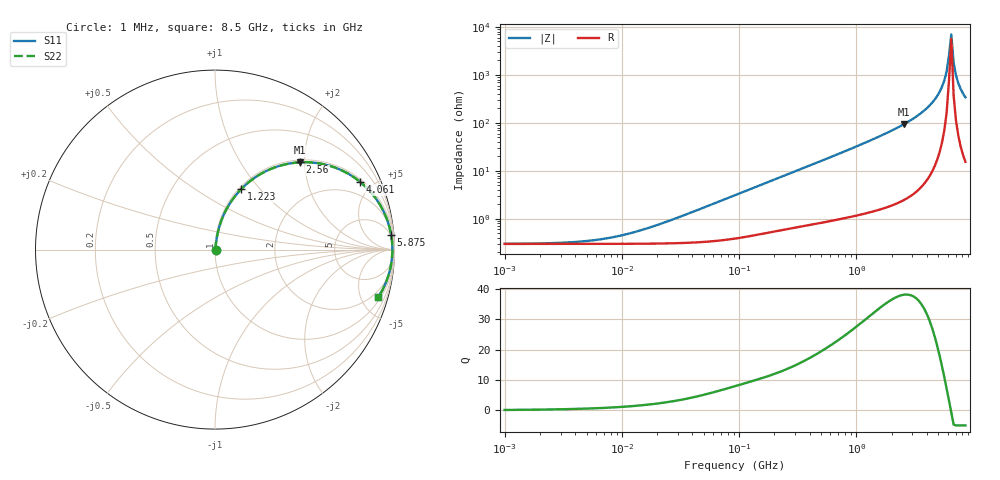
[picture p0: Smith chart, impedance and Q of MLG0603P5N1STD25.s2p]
! S-Parameter Data Generated by TDK Corporation
! Copyright(C) 2025 TDK Corporation.
! All Rights Reserved.
! TDK P/N: MLG0603P5N1STD25 (SMD / SMT Inductor (Coil))
! Property: L=5.1nH at 500MHz
! Size(LxWxT): 0.6x0.3x0.3mm
! Model Type: s2p (Touchstone File Format Version 1.0)
! Frequency: DC=Yes Start=1MHz Stop=8500MHz 198points Log-sweep
! Model Generated on Feb. 6, 2025
! Terms and conditions regarding TDK Simulation Models:
! 1)This simulation model is being provided solely for informational
!  purposes. Please refer to the specifications of the products in
!  terms of detailed characteristics of such products.
! 2)In no event shall TDK Corporation of any of its subsidiaries be
!  liable for any loss or damage arising, directly or indirectly,
!  from any information contained in this simulation model, including,
!  but not limited to loss or damages arising from any inaccuracies,
!  omissions or errors in connection with such information.
! 3)Any and all copyrights on this simulation model are owned by
!  TDK Corporation.  Duplication or redistribution of this simulation
!  model without prior written permission from TDK Corporation
!  is prohibited.
! 4)This simulation model is subject to any modification or change
!  without any prior notice.
! 5)Neither TDK Corporation nor any of its subsidiaries shall make any
!  warranty, express or implied, including but not limited to the
!  correctness, implied warranties of merchantability and fitness for
!  a particular purpose with respect to this simulation models.
! 6)The use of this simulation model shall be deemed to have consented
!  to the terms and conditions hereof.
! Port Assignments:
!  1 ---@@@--- 2
! Applicable Conditions:
!  Temperature = 25 degC
!  DC Bias Current = 0 A
!  Small Signal Operation
# Hz S MA R 50
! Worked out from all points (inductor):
!   197 points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, 1 MHz to 8.5 GHz, reference 50 ohm
!   read as one part in series: L = 5.38 nH near 27.76 MHz
!   highest Q = 38.1 at 2.56 GHz (marker M1), where L = 5.89 nH
!   self-resonance near 6.153 GHz
!   S11 on the Smith chart (normalised r, x): 1 MHz: 1.01, +0.00; 1.223 GHz: 1.03, +0.80; 2.56 GHz: 1.05, +1.90; 4.061 GHz: 1.14, +4.22; 5.875 GHz: 4, +23; 8.5 GHz: 1.31, -6.81
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1000000  0.00301 6.4  0.997 -0.0  0.997 -0.0  0.00301 6.4
4587603  0.003372 27.3  0.997 -0.1  0.997 -0.1  0.003372 27.3
9601846  0.004421 47.0  0.997 -0.2  0.997 -0.2  0.004421 47.0
2.10461e7  0.007733 66.4  0.9969 -0.4  0.9969 -0.4  0.007733 66.4
9.219544e7  0.03095 81.1  0.9957 -1.8  0.9957 -1.8  0.03095 81.1
4.229561e8  0.1338 79.1  0.9835 -7.7  0.9835 -7.7  0.1338 79.1
7.707615e8  0.2377 73.9  0.9616 -13.7  0.9616 -13.7  0.2377 73.9
1.222927e9  0.3658 66.7  0.9187 -21.4  0.9187 -21.4  0.3658 66.7
1.940355e9  0.5476 55.2  0.8217 -33.2  0.8217 -33.2  0.5476 55.2
2.559585e9  0.6792 45.7  0.7164 -42.8  0.7164 -42.8  0.6792 45.7
3.224109e9  0.7917 36.1  0.5899 -52.3  0.5899 -52.3  0.7917 36.1
4.061159e9  0.8926 25.0  0.4229 -63.1  0.4229 -63.1  0.8926 25.0
4.664383e9  0.9401 17.7  0.3043 -69.9  0.3043 -69.9  0.9401 17.7
5.115526e9  0.9638 12.6  0.2189 -74.2  0.2189 -74.2  0.9638 12.6
5.610304e9  0.9799 7.4  0.1299 -77.4  0.1299 -77.4  0.9799 7.4
5.87536e9  0.9849 4.8  0.08461 -77.3  0.08461 -77.3  0.9849 4.8
6.152938e9  0.9877 2.2  0.03956 -70.9  0.03956 -70.9  0.9877 2.2
6.44363e9  0.9884 -0.5  0.01421 35.3  0.01421 35.3  0.9884 -0.5
6.748056e9  0.987 -3.1  0.05566 74.9  0.05566 74.9  0.987 -3.1
7.066863e9  0.9833 -5.8  0.101 77.6  0.101 77.6  0.9833 -5.8
7.750377e9  0.9697 -11.0  0.191 75.4  0.191 75.4  0.9697 -11.0
8.5e9  0.9481 -16.1  0.278 71.3  0.278 71.3  0.9481 -16.1
